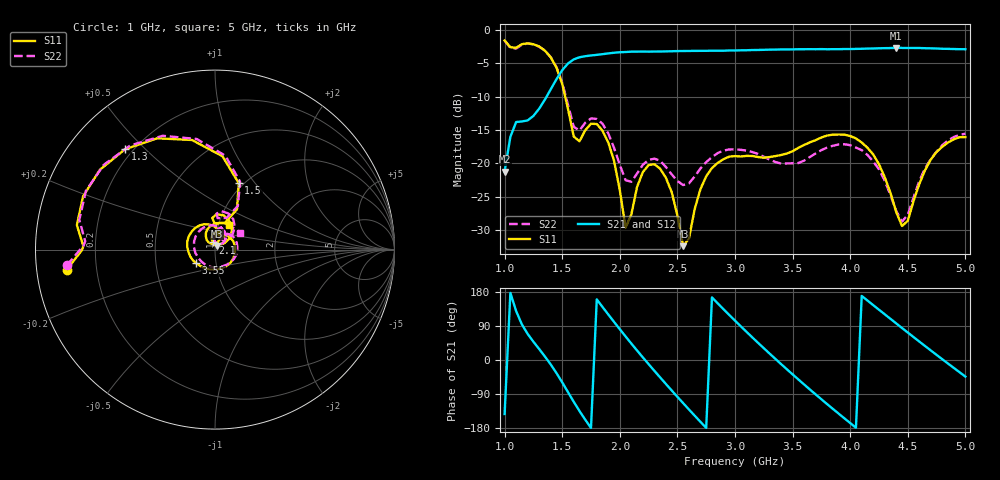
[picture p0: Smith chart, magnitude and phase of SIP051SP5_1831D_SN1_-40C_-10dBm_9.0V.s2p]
# GHz  S  dB  R  50
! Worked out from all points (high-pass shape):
!   81 points, 1 GHz to 5 GHz, reference 50 ohm
!   highest |S21| = -2.69 dB at 4.4 GHz (marker M1); lowest = -21.3 dB at 1 GHz (marker M2)
!   |S21| within 3 dB of the highest: 1.518 GHz to end of sweep
!   lowest |S11| = -32.4 dB at 2.55 GHz (marker M3), VSWR 1.05, Z = 51.2 + j2.1 ohm
!   |S11| at or under -10 dB: 1.525 GHz to end of sweep
!   |S22| runs from -28.7 to -1.6 dB; largest |S21 - S12| = 0.0017
!   S11 on the Smith chart (normalised r, x): 1 GHz: 0.09, -0.07; 1.3 GHz: 0.17, +0.44; 1.5 GHz: 0.95, +0.83; 2.1 GHz: 0.98, +0.08; 3.55 GHz: 0.80, -0.12; 5 GHz: 1.12, +0.32
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1  -1.58 -172.3  -21.25 -142.6  -21.29 -142.5  -1.62 -174.0
1.1  -2.69 178.5  -13.82 129.2  -13.84 129.3  -2.80 176.4
1.3  -2.49 131.9  -11.81 29.0  -11.80 28.9  -2.52 129.2
1.5  -8.11 70.3  -6.05 -59.0  -6.04 -59.0  -7.91 69.6
1.6  -16.00 69.6  -4.42 -110.2  -4.41 -110.2  -14.53 69.9
1.7  -15.06 95.1  -3.95 -157.6  -3.95 -157.5  -13.92 87.3
1.9  -16.89 48.5  -3.53 120.1  -3.53 120.1  -15.53 48.7
2.05  -29.65 60.3  -3.32 62.2  -3.31 62.2  -22.54 50.8
2.1  -27.70 105.2  -3.26 43.4  -3.27 43.5  -22.78 67.3
2.35  -20.82 61.7  -3.24 -46.0  -3.23 -46.0  -19.62 53.6
2.55  -32.44 59.0  -3.17 -113.9  -3.15 -113.9  -23.27 52.4
2.75  -21.96 86.4  -3.14 -179.2  -3.13 -179.1  -19.84 58.4
3  -18.93 9.4  -3.09 103.9  -3.07 103.8  -17.93 17.5
3.3  -19.07 -84.6  -2.96 17.1  -2.97 17.0  -19.45 -52.2
3.55  -17.69 -144.7  -2.90 -51.3  -2.90 -51.4  -19.97 -135.9
3.7  -16.53 -175.9  -2.90 -90.8  -2.89 -90.8  -18.53 172.9
4.05  -16.28 112.6  -2.85 -178.6  -2.84 -178.7  -17.65 83.8
4.35  -24.47 66.0  -2.73 108.5  -2.73 108.5  -24.81 39.4
4.4  -27.35 69.8  -2.69 96.4  -2.70 96.4  -27.20 45.1
4.5  -28.64 120.5  -2.71 72.4  -2.70 72.5  -27.74 86.4
4.7  -19.43 118.1  -2.77 25.1  -2.76 25.1  -19.37 86.5
5  -16.08 61.3  -2.90 -43.8  -2.91 -43.9  -15.58 33.8
